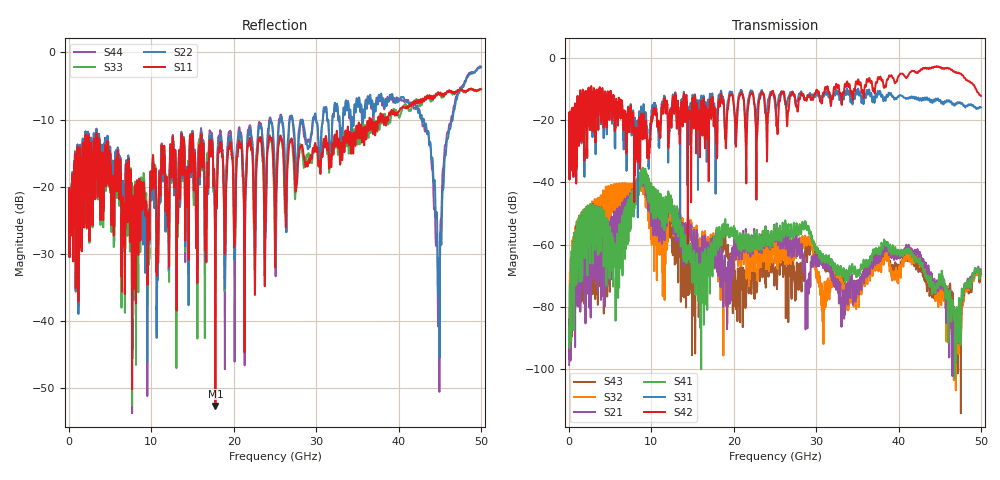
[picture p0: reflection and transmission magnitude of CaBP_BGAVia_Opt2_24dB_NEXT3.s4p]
!* Samtec Inc. NovaRay Examax Flyover System  *
!*  REV DATE  = 08/08/18  *
!*  TYPE  = TOUCHSTONE  *
!*  PORTS  = 4 port  *
!*  UNITS  = GHz  *
!*  DATA RANGE = DC  to 50 GHz; 10 MHz Step  *
!*  PARAMETER  = S  *
!*  FORMAT  = Real-Imaginary  *
!*  REFERENCE  = 50 ohms  *
!*  SOURCE  = HFSS  *
!*  VALIDATED  = No  *
!*  MANUFACTURER = SAMTEC  *
!*  INTERCONNECT = NVAx to EBCx to EBCx to NVAx  *
!*  [Full Channel NVAx to EBCx to EBCx to NVAx  with PCB Trace and BGA Via]  *
!*  BOUNDARY A  = Silicon BGA Ball Pad  *
!*  BOUNDARY B  = Silicon BGA Ball Pad  *
!*  NVAx (end a) ->>- (end b) NVAx  *
!*  Port 01 ->>- Port 02  *
!*  Port 03 ->>- Port 04  *
!***************************** CHANNEL MODEL ******************************************
# GHz S RI R 50
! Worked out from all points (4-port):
!   5000 points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, 10 MHz to 50 GHz, reference 50 ohm
!   strongest paths, dB at 10 MHz, 12.51 GHz, 25.01 GHz, 37.51 GHz, 50 GHz:
!     S42: -23.1, -15.3, -13.0, -6.3, -12.3
!     S31: -23.2, -14.5, -15.2, -10.7, -16.0
!     S41: -89.9, -50.0, -56.4, -62.3, -68.4
!     S21: -98.6, -49.7, -57.0, -65.3, -67.9
!     S32: -90.6, -49.6, -63.0, -67.0, -69.0
!     S43: -95.7, -60.7, -67.9, -63.9, -69.3
!   lowest |S11| = -52.7 dB at 17.77 GHz (marker M1), VSWR 1.00, Z = 49.8 - j0.145 ohm
!   |S11| at or under -10 dB: start of sweep to 36.46 GHz; 36.55 GHz to 36.75 GHz (204 MHz wide, 0.557 % of centre); 36.79 GHz to 37.51 GHz (722.9 MHz wide, 1.95 % of centre)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
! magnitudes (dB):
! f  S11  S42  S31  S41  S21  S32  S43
! 10 MHz  -22.7  -23.1  -23.2  -89.9  -98.6  -90.6  -95.7
! 8.84 GHz  -20.1  -20.1  -18.1  -36.2  -37.6  -40.9  -36.8
! 15.17 GHz  -18.8  -19.3  -17.3  -62.0  -55.3  -54.8  -63.9
! 17.77 GHz  -52.7  -21.4  -28.1  -63.1  -65.8  -66.1  -63.6
! 41.05 GHz  -8.2  -6.2  -12.9  -61.6  -60.5  -61.8  -64.0
! 44.79 GHz  -6.0  -3.0  -13.1  -73.9  -74.4  -78.9  -76.3
! 50 GHz  -5.5  -12.3  -16.0  -68.4  -67.9  -69.0  -69.3
